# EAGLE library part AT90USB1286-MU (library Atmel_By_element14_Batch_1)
Microcontroller
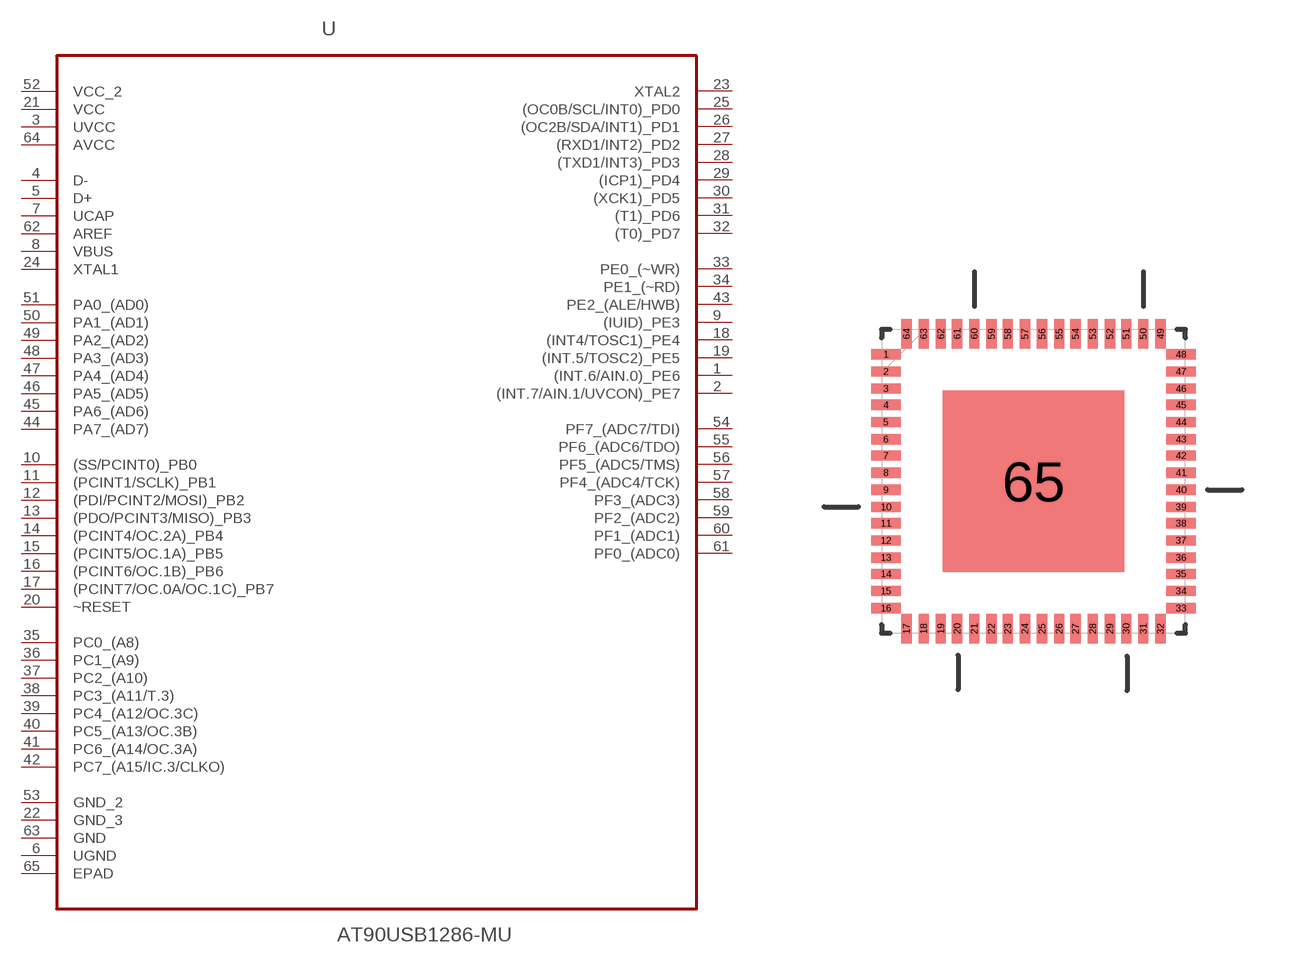
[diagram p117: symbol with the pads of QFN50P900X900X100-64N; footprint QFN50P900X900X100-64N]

Designator prefix U

## AT90USB1286-MU (DESCRIPTION: Microcontroller; MPN: AT90USB1286-MU; OC_FARNELL: 1841598; OC_NEWARK: 12T1384; PACKAGE: QFN-64; SUPPLIER: ATMEL)  [QFN50P900X900X100-64N]
1  (INT.6/AIN.0)_PE6
2  (INT.7/AIN.1/UVCON)_PE7
3  UVCC  pwr
4  D-  in
5  D+  in
6  UGND  pas
7  UCAP  pas
8  VBUS  pas
9  (IUID)_PE3
10  (SS/PCINT0)_PB0
11  (PCINT1/SCLK)_PB1
12  (PDI/PCINT2/MOSI)_PB2
13  (PDO/PCINT3/MISO)_PB3
14  (PCINT4/OC.2A)_PB4
15  (PCINT5/OC.1A)_PB5
16  (PCINT6/OC.1B)_PB6
17  (PCINT7/OC.0A/OC.1C)_PB7
18  (INT4/TOSC1)_PE4
19  (INT.5/TOSC2)_PE5
20  ~RESET  in
21  VCC  pwr
22  GND_3  pas
23  XTAL2  out
24  XTAL1  in
25  (OC0B/SCL/INT0)_PD0
26  (OC2B/SDA/INT1)_PD1
27  (RXD1/INT2)_PD2
28  (TXD1/INT3)_PD3
29  (ICP1)_PD4
30  (XCK1)_PD5
31  (T1)_PD6
32  (T0)_PD7
33  PE0_(~WR)
34  PE1_(~RD)
35  PC0_(A8)
36  PC1_(A9)
37  PC2_(A10)
38  PC3_(A11/T.3)
39  PC4_(A12/OC.3C)
40  PC5_(A13/OC.3B)
41  PC6_(A14/OC.3A)
42  PC7_(A15/IC.3/CLKO)
43  PE2_(ALE/HWB)
44  PA7_(AD7)
45  PA6_(AD6)
46  PA5_(AD5)
47  PA4_(AD4)
48  PA3_(AD3)
49  PA2_(AD2)
50  PA1_(AD1)
51  PA0_(AD0)
52  VCC_2  pwr
53  GND_2  pas
54  PF7_(ADC7/TDI)
55  PF6_(ADC6/TDO)
56  PF5_(ADC5/TMS)
57  PF4_(ADC4/TCK)
58  PF3_(ADC3)
59  PF2_(ADC2)
60  PF1_(ADC1)
61  PF0_(ADC0)
62  AREF  in
63  GND  pas
64  AVCC  pwr
65  EPAD  pas

## Footprint QFN50P900X900X100-64N (pad centres in mm)
smd 0.864 x 0.305: 1 -4.369,3.759; 2 -4.369,3.251; 3 -4.369,2.743; 4 -4.369,2.261; 5 -4.369,1.753; 6 -4.369,1.245; 7 -4.369,0.762; 8 -4.369,0.254; 9 -4.369,-0.254; 10 -4.369,-0.762; 11 -4.369,-1.245; 12 -4.369,-1.753; 13 -4.369,-2.261; 14 -4.369,-2.743; 15 -4.369,-3.251; 16 -4.369,-3.759; 33 4.369,-3.759; 34 4.369,-3.251; 35 4.369,-2.743; 36 4.369,-2.261; 37 4.369,-1.753; 38 4.369,-1.245; 39 4.369,-0.762; 40 4.369,-0.254; 41 4.369,0.254; 42 4.369,0.762; 43 4.369,1.245; 44 4.369,1.753; 45 4.369,2.261; 46 4.369,2.743; 47 4.369,3.251; 48 4.369,3.759
smd 0.305 x 0.864: 17 -3.759,-4.369; 18 -3.251,-4.369; 19 -2.743,-4.369; 20 -2.261,-4.369; 21 -1.753,-4.369; 22 -1.245,-4.369; 23 -0.762,-4.369; 24 -0.254,-4.369; 25 0.254,-4.369; 26 0.762,-4.369; 27 1.245,-4.369; 28 1.753,-4.369; 29 2.261,-4.369; 30 2.743,-4.369; 31 3.251,-4.369; 32 3.759,-4.369; 49 3.759,4.369; 50 3.251,4.369; 51 2.743,4.369; 52 2.261,4.369; 53 1.753,4.369; 54 1.245,4.369; 55 0.762,4.369; 56 0.254,4.369; 57 -0.254,4.369; 58 -0.762,4.369; 59 -1.245,4.369; 60 -1.753,4.369; 61 -2.261,4.369; 62 -2.743,4.369; 63 -3.251,4.369; 64 -3.759,4.369
smd 5.385 x 5.385: 65 0,0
